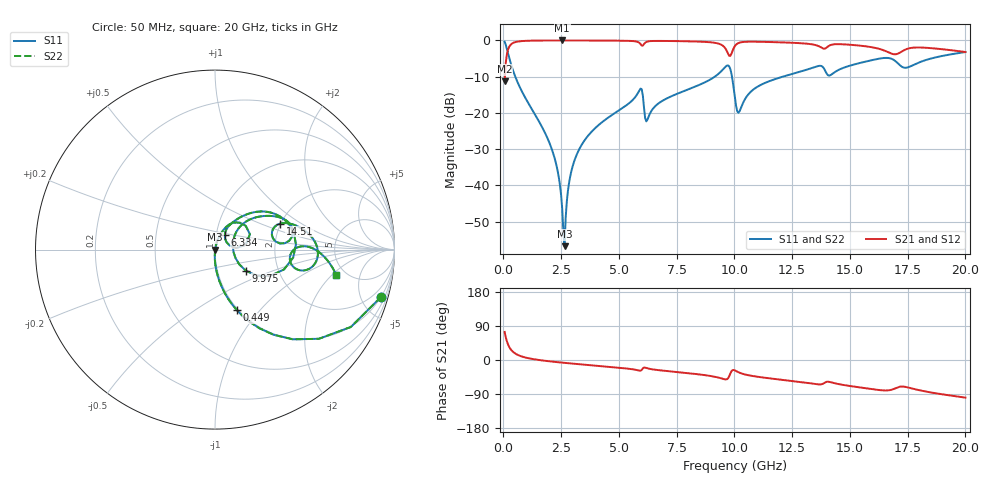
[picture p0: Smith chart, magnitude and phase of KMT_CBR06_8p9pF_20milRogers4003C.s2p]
! Data measured by Modelithics Inc. support@modelithics.com 813-866-6335
! KEMET CBR0603 8.9pF, Pad Width= 0.851mm, Pad Length= 0.64mm, Pad Gap= 0.62mm, 20mil Rogers 4003C substrate Data, January 2022
# hz S ma R 50
! 2 Port Network Data from SP1.SP block
! freq  magS11  angS11  magS21  angS21  magS12  angS12  magS22  angS22
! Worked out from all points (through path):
!   401 points, 50 MHz to 20 GHz, reference 50 ohm
!   highest |S21| = -0.01 dB at 2.544 GHz (marker M1); lowest = -11.3 dB at 50 MHz (marker M2)
!   group delay of S21, straight-line fit = 14.5 ps
!   lowest |S11| = -56.8 dB at 2.643 GHz (marker M3), VSWR 1.00, Z = 50.1 + j0.0531 ohm
!   |S11| at or under -10 dB: 512.5 MHz to 9.151 GHz (8.638 GHz wide, 179 % of centre); 9.893 GHz to 12.09 GHz (2.202 GHz wide, 20 % of centre)
!   |S22| runs from -56.8 to -0.3 dB; largest |S21 - S12| = 0
!   S11 on the Smith chart (normalised r, x): 50 MHz: 0.99, -7.03; 449 MHz: 0.98, -0.76; 6.334 GHz: 1.10, +0.18; 9.975 GHz: 1.37, -0.34; 14.51 GHz: 1.99, +0.68; 20 GHz: 4.17, -2.28
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5e7  0.9624 -15.9  0.2713 74.1  0.2713 74.1  0.9624 -15.9
4.49e8  0.3582 -70.2  0.9328 19.7  0.9328 19.7  0.3582 -70.2
2.094875e9  0.03153 -92.1  0.9983 -4.2  0.9983 -4.2  0.03153 -92.1
2.394125e9  0.01307 -90.7  0.9986 -6.1  0.9986 -6.1  0.01307 -90.7
2.54375e9  0.004798 -81.9  0.9987 -7.0  0.9987 -7.0  0.004798 -81.9
2.6435e9  0.001452 21.4  0.9986 -7.6  0.9986 -7.6  0.001452 21.4
2.94275e9  0.01582 75.9  0.9984 -9.3  0.9984 -9.3  0.01582 75.9
3.391625e9  0.03655 76.0  0.9978 -11.7  0.9978 -11.7  0.03655 76.0
5.885375e9  0.2051 46.6  0.9259 -28.1  0.9259 -28.1  0.2051 46.6
6.184625e9  0.0765 32.7  0.9527 -21.1  0.9527 -21.1  0.0765 32.7
6.33425e9  0.09668 55.8  0.9772 -23.4  0.9772 -23.4  0.09668 55.8
6.73325e9  0.1368 60.4  0.984 -26.9  0.984 -26.9  0.1368 60.4
9.675875e9  0.4492 11.7  0.7093 -50.8  0.7093 -50.8  0.4492 11.7
9.975125e9  0.2103 -34.3  0.7909 -26.5  0.7909 -26.5  0.2103 -34.3
1.0025e10  0.159 -31.4  0.841 -27.7  0.841 -27.7  0.159 -31.4
1.02245e10  0.1056 18.8  0.9317 -33.6  0.9317 -33.6  0.1056 18.8
1.10225e10  0.2322 42.1  0.9585 -44.4  0.9585 -44.4  0.2322 42.1
1.336662e10  0.4172 24.3  0.8825 -62.1  0.8825 -62.1  0.4172 24.3
1.451375e10  0.3924 21.7  0.8881 -63.7  0.8881 -63.7  0.3924 21.7
1.670825e10  0.5691 -6.1  0.6766 -79.8  0.6766 -79.8  0.5691 -6.1
1.74065e10  0.4194 -5.7  0.7487 -71.0  0.7487 -71.0  0.4194 -5.7
2e10  0.691 -11.9  0.6914 -99.3  0.6914 -99.3  0.691 -11.9
